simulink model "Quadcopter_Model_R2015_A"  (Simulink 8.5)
settings: Solver=ode45  SolverMode=SingleTasking  StartTime=0.0  StopTime=runtime  RelTol=1e-3
InitFcn:
  | clear mex
  | delete test_model_sfun.mexw64
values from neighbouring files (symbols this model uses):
  g = 9.81    [modelParameters.m]    (also in analyzeIMU_data.m = 9.8; getMomentOfInertia.m = 9.80665)
  height_controlled_o = dataStruct.RC_Throttle_Constant.data(1)    [modelParameters.m]
  If = 0.3836    [modelParameters.m]    (also in thrustDragConstantCalculations.m = [If0; If1; If2; If3]; Kd_error.m = I_0 * sign(rotor_speed_0) + I_1 * rotor_speed_0 + I_2 * roto)
  Jreq = 4.2012e-05    [modelParameters.m]
  Jxx = 0.0130    (= 0.013)    [modelParameters.m]
  Jyy = 0.0140    (= 0.014)    [modelParameters.m]
  Jzz = 0.0285    [modelParameters.m]
  Kd = 1.4852e-07    [modelParameters.m]    (also in calcDragConstant.m = ((A'*A)^-1)*A'*b; thrustDragConstantCalculations.m = calcDragConstant(data, Pmin, Pmax, Rm, Kv, Kq, If); Kd_error.m = 1.0317e-07)
  Kq = 96.3422    [modelParameters.m]    (also in thrustDragConstantCalculations.m; Kd_error.m)
  Kt = 1.2007e-05    [modelParameters.m]    (also in calcThrustConstant.m = ((A'*A)^(-1))*(A'*T); thrustDragConstantCalculations.m = calcThrustConstant(data))
  Kv = 96.3422    [modelParameters.m]    (also in thrustDragConstantCalculations.m; Kd_error.m)
  m = 1.140    (= 1.14)    [modelParameters.m]
  omega0_o = (sqrt(((height_controlled_o      - Pmin)/(Pmax - Pmin)* Vb - Rm * If) * 4 *      Rm * Kv^2 * Kq * Kd + 1) - 1) / (2 * Rm *       Kv * Kq * Kd)    [modelParameters.m]
  omega1_o = omega0_o    [modelParameters.m]
  omega2_o = omega0_o    [modelParameters.m]
  omega3_o = omega0_o    [modelParameters.m]
  pitch_o = pitch_measured_VRPN(1)    [modelParameters.m]
  pitchrate_o = (pitch_measured_VRPN(1) - pitch_measured_VRPN(2))/(time(1) - time(2))    [modelParameters.m]
  Pmax = 2e5    (= 200000)    [modelParameters.m]    (also in thrustDragConstantCalculations.m; Kd_error.m)
  Pmin = 1e5    (= 100000)    [modelParameters.m]    (also in thrustDragConstantCalculations.m; Kd_error.m)
  rhx = 0.16    [modelParameters.m]
  rhy = 0.16    [modelParameters.m]
  rhz = 0.03    [modelParameters.m]
  Rm = 0.2308    [modelParameters.m]    (also in thrustDragConstantCalculations.m; Kd_error.m)
  roll_o = roll_measured_VRPN(1)    [modelParameters.m]
  rollrate_o = (roll_measured_VRPN(1) - roll_measured_VRPN(2))/(time(1) - time(2))    [modelParameters.m]
  Tc = 0.04    [modelParameters.m]
  Tq = 0.005    [modelParameters.m]
  Vb = 11.4    [modelParameters.m]    (also in calcDragConstant.m = [data.(6); data.(6); data.(6); data.(6)]; Kd_error.m = data.(6))
  x_controlled_o = 0    [modelParameters.m]
  x_o = x_position(1)    [modelParameters.m]
  x_vel_o = (x_position(1) - x_position(2))/(time(1) - time(2))    [modelParameters.m]
  y_controlled_o = 0    [modelParameters.m]
  y_o = y_position(1)    [modelParameters.m]
  y_vel_o = (y_position(1) - y_position(2))/(time(1) - time(2))    [modelParameters.m]
  yaw_controlled_o = 0    [modelParameters.m]
  yaw_o = 0    [modelParameters.m]
  yawrate_o = 0    [modelParameters.m]
  z_o = z_position(1)    [modelParameters.m]
  z_vel_o = (z_position(1) - z_position(2))/(time(1) - time(2))    [modelParameters.m]
undefined symbols (not defined in the file or in its folder): DiscIntNeverNeededParam
libraries: simulink x12, vrlib x2
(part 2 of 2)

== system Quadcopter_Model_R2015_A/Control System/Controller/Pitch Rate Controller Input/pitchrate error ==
  From Workspace2 : FromWorkspace  VariableName=pitchrate_error  SampleTime=Tq
  pitchrate_error : Outport
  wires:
  From Workspace2/1 -> pitchrate_error/1

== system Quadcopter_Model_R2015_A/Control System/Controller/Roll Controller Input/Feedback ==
  roll_error_model : Inport
  roll_error : Outport
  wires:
  roll_error_model/1 -> roll_error/1

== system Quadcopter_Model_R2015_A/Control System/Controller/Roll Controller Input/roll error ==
  From Workspace4 : FromWorkspace  VariableName=roll_error  SampleTime=Tq
  roll_error : Outport
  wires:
  From Workspace4/1 -> roll_error/1

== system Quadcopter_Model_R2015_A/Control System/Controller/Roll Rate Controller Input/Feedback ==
  rollrate_error_model : Inport
  rollrate_error : Outport
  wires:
  rollrate_error_model/1 -> rollrate_error/1

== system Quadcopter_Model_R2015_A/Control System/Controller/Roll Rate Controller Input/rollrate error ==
  From Workspace5 : FromWorkspace  VariableName=rollrate_error  SampleTime=Tq
  rollrate_error : Outport
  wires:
  From Workspace5/1 -> rollrate_error/1

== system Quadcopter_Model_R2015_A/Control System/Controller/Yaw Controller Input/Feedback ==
  yaw_error_model : Inport
  yaw_error : Outport
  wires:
  yaw_error_model/1 -> yaw_error/1

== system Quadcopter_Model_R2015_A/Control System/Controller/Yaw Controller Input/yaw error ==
  From Workspace7 : FromWorkspace  VariableName=yaw_error  SampleTime=Tc
  yaw_error : Outport
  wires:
  From Workspace7/1 -> yaw_error/1

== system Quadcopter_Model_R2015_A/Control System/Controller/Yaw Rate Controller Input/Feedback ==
  yawrate_error_model : Inport
  yawrate_error : Outport
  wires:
  yawrate_error_model/1 -> yawrate_error/1

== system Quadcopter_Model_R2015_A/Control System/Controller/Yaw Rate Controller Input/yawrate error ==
  From Workspace8 : FromWorkspace  VariableName=yawrate_error  SampleTime=Tq
  yawrate_error : Outport
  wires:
  From Workspace8/1 -> yawrate_error/1

== matlab function Actuation/Gravity

 ==
function E_Fg = gravity(m, g)

E_Fg = [0; 0; m*g];

== matlab function Actuation/Lbe





 ==
function E_ro  = linear_body_earth_conversion(B_vo, euler_angles)

euler_rates = zeros(3,1);
E_ro = zeros(3,1);

phi = euler_angles(1);
theta = euler_angles(2);
psi = euler_angles(3);

Leb = [cos(theta)*cos(psi), sin(phi)*sin(theta)*cos(psi)-cos(phi)*sin(psi), cos(phi)*sin(theta)*cos(psi)+sin(phi)*sin(psi); ...
       cos(theta)*sin(psi), sin(phi)*sin(theta)*sin(psi)+cos(phi)*cos(psi), cos(phi)*sin(theta)*sin(psi)-sin(phi)*cos(psi); ...
           -sin(theta)    ,                sin(phi)*cos(theta)            ,                 cos(phi)*cos(theta)           ];

E_ro = Leb * B_vo;

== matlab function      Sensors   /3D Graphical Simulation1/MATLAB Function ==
function y = eigenaxis_ucart(u)


if abs(u(1))< 0.0001
    u(1) = 0.0001;
end

if abs(u(2))< 0.0001
    u(2) = 0.0001;
end

if abs(u(3))< 0.0001
    u(3) = 0.0001;
end

u = [ -u(1); -u(2); u(3) ];% [Pitch, Yaw, Roll] 

C11 = cos(u(2))*cos(u(3));
C12 = cos(u(2))*sin(u(3));
C13 = -sin(u(2));
C21 = sin(u(1))*sin(u(2))*cos(u(3))-cos(u(1))*sin(u(3));
C22 = sin(u(1))*sin(u(2))*sin(u(3))+cos(u(1))*cos(u(3));
C23 = sin(u(1))*cos(u(2));
C31 = cos(u(1))*sin(u(2))*cos(u(3))+sin(u(1))*sin(u(3));
C32 = cos(u(1))*sin(u(2))*sin(u(3))-sin(u(1))*cos(u(3));
C33 = cos(u(1))*cos(u(2));
    
theta = acos(0.5*(C11+C22+C33-1));

e = [C23-C32; C31-C13; C12-C21]/(2*sin(theta));
    
y = [e; theta];

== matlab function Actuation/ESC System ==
function Vb_eff   = ESC(P, Pmin, Pmax, Vb)

P1 = P(1);
P2 = P(2);
P3 = P(3);
P4 = P(4);

% Define u_Pi for each of the rotors, limiting it to be greater than 0
% u_P0 = (rotor_0_duty_cycle/100 - Pmin) / (Pmax - Pmin);
% u_P1 = (rotor_1_duty_cycle/100 - Pmin) / (Pmax - Pmin);
% u_P2 = (rotor_2_duty_cycle/100 - Pmin) / (Pmax - Pmin);
% u_P3 = (rotor_3_duty_cycle/100 - Pmin) / (Pmax - Pmin);
u_P0 = (P1 - Pmin) / (Pmax - Pmin);
u_P1 = (P2 - Pmin) / (Pmax - Pmin);
u_P2 = (P3 - Pmin) / (Pmax - Pmin);
u_P3 = (P4 - Pmin) / (Pmax - Pmin);


% Determine the effective battery voltage from each ESC
Vb_eff_0 = u_P0 * Vb;
Vb_eff_1 = u_P1 * Vb;
Vb_eff_2 = u_P2 * Vb;
Vb_eff_3 = u_P3 * Vb;
    
Vb_eff = [Vb_eff_0, Vb_eff_1, Vb_eff_2, Vb_eff_3];

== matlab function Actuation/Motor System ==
function w_dot = motor(Vb_eff, w, Rm, Kv, Kq, Kd, If, Jreq)

% Define each motors effective battery voltage
Vb_eff_0 = Vb_eff(1);
Vb_eff_1 = Vb_eff(2);
Vb_eff_2 = Vb_eff(3);
Vb_eff_3 = Vb_eff(4);

% Determine the angular velocity of each rotor from feedback
w_0 = w(1);
w_1 = w(2);
w_2 = w(3);
w_3 = w(4);

% Determine angular acceleration of each rotor
w_0_dot = 1/(Jreq*Rm*Kq) * Vb_eff_0 - 1/(Jreq*Rm*Kq*Kv) * w_0 - 1/(Jreq*Kq)*If - (Kd/Jreq) * w_0^2;
w_1_dot = 1/(Jreq*Rm*Kq) * Vb_eff_1 - 1/(Jreq*Rm*Kq*Kv) * w_1 - 1/(Jreq*Kq)*If - (Kd/Jreq) * w_1^2;
w_2_dot = 1/(Jreq*Rm*Kq) * Vb_eff_2 - 1/(Jreq*Rm*Kq*Kv) * w_2 - 1/(Jreq*Kq)*If - (Kd/Jreq) * w_2^2;
w_3_dot = 1/(Jreq*Rm*Kq) * Vb_eff_3 - 1/(Jreq*Rm*Kq*Kv) * w_3 - 1/(Jreq*Kq)*If - (Kd/Jreq) * w_3^2;

w_dot = [w_0_dot, w_1_dot, w_2_dot, w_3_dot];

== matlab function Actuation/Rotor System







 ==
function [B_omega_dot, B_vo_dot]= rotor(w_dot, w, B_Fg, B_omega, B_vo, m, Kt, Kd, rhx, rhy, rhz, Jreq, Jxx, Jyy, Jzz)

% Create J vector
J = [Jxx,  0 ,  0 ; ...
      0 , Jyy,  0 ; ...
      0 ,  0 , Jzz;];

% Create r_hi vector
rh_0 = [-rhx; rhy; -rhz];
rh_1 = [rhx; rhy; -rhz];
rh_2 = [-rhx; -rhy; -rhz];
rh_3 = [rhx; -rhy; -rhz];

% Define vector from body frame origin to center of mass
br_oc = [0; 0; 0];

% Define 3x3 Identity Matrix
I = eye(3);

% Create gamma vectors
gamma_Ti = [0; 0; -1];
gamma_omega_03 = [0; 0; 1];  %Rotors 0 and 3 use this gamma_omega vector
gamma_omega_12 = [0; 0; -1]; %Rotors 1 and 2 use this gamma_omega vector

% Define angular velocities for each rotor
w_0 = w(1);
w_1 = w(2);
w_2 = w(3);
w_3 = w(4);

% Define angular acceleration for each rotor
w_0_dot = w_dot(1);
w_1_dot = w_dot(2);
w_2_dot = w_dot(3);
w_3_dot = w_dot(4);

% Define the rotor force in the z-direction from each rotor
B_Fr_0 = Kt * w_0 * w_0 * gamma_Ti;
B_Fr_1 = Kt * w_1 * w_1 * gamma_Ti;
B_Fr_2 = Kt * w_2 * w_2 * gamma_Ti;
B_Fr_3 = Kt * w_3 * w_3 * gamma_Ti;

% Sum up the rotor forces in the z-direction from each vector to get the
% total body force in the z-direction
B_Fr = B_Fr_0 + B_Fr_1 + B_Fr_2 + B_Fr_3;

% Define the in-plane drag and induced torque produced by each rotor
 B_Q_d0 = -1 * Kd * w_0 * w_0 * gamma_omega_03;
 B_Q_d1 = -1 * Kd * w_1 * w_1 * gamma_omega_12;
 B_Q_d2 = -1 * Kd * w_2 * w_2 * gamma_omega_12;
 B_Q_d3 = -1 * Kd * w_3 * w_3 * gamma_omega_03;

% Sum up the total in-plane drag and induced torque to get the total
% in-plane drag and induced torque on the body
B_Q_d = B_Q_d0 + B_Q_d1 + B_Q_d2 + B_Q_d3;

% Define the force lever arm torque created from the force produced by each
% rotor in the z-direction
B_Q_F0 = cross( rh_0, B_Fr_0 );
B_Q_F1 = cross( rh_1, B_Fr_1 );
B_Q_F2 = cross( rh_2, B_Fr_2 );
B_Q_F3 = cross( rh_3, B_Fr_3 );

B_Q_F = B_Q_F0 + B_Q_F1 + B_Q_F2 + B_Q_F3;

%Define the change in angular momentum torque produced by each rotor 
B_Q_L0 = -1 * Jreq * ( cross(B_omega, w_0 * gamma_omega_03) + w_0_dot * gamma_omega_03 );
B_Q_L1 = -1 * Jreq * ( cross(B_omega, w_1 * gamma_omega_12) + w_1_dot * gamma_omega_12 ); 
B_Q_L2 = -1 * Jreq * ( cross(B_omega, w_2 * gamma_omega_12) + w_2_dot * gamma_omega_12 ); 
B_Q_L3 = -1 * Jreq * ( cross(B_omega, w_3 * gamma_omega_03) + w_3_dot * gamma_omega_03 );

% Sum up the total change in angular momentum torque produced by each rotor
B_Q_L = B_Q_L0 + B_Q_L1 + B_Q_L2 + B_Q_L3;

% Define the total rotor system torque as the sum of the in-plane drag and
% induced torque, force lever arm torque, and change in angular momentum
% torques
B_Q = B_Q_d + B_Q_F + B_Q_L;

% Define the body forces in the z-direction from each vector to get the
% total body force in the z-direction
B_F = B_Fr + B_Fg; 

% Define the body frame linear velocities
B_vo_dot = (m*I)^(-1) * ( B_F - cross( B_omega, m*(B_vo + cross(B_omega, br_oc)) ) );

% Define the body frame angular velocities
B_omega_dot = J ^(-1) * ( B_Q - cross(B_omega, J * B_omega) - cross(br_oc, B_F) );

== matlab function Actuation/Aeb














 ==
function euler_rates = angular_body_earth_conversion(B_omega, euler_angles)

phi = euler_angles(1);
theta = euler_angles(2);

Aeb = [1,  sin(phi)*tan(theta), cos(phi)*tan(theta); ...
       0,      cos(phi)       ,        -sin(phi)   ; ...
       0,  sin(phi)/cos(theta), cos(phi)/cos(theta)];

   
euler_rates = Aeb * B_omega;

== matlab function Actuation/Lbe

















 ==
function [B_Fg, B_g]  = linear_earth_body_conversion(E_Fg, euler_angles, m)

phi = euler_angles(1);
theta = euler_angles(2);
psi = euler_angles(3);

Lbe = [             cos(theta)*cos(psi)              ,          cos(theta)*sin(psi)                  ,     -sin(theta)    ; ...
       sin(phi)*sin(theta)*cos(psi)-cos(phi)*sin(psi), sin(phi)*sin(theta)*sin(psi)+cos(phi)*cos(psi), sin(phi)*cos(theta); ...
       cos(phi)*sin(theta)*cos(psi)+sin(phi)*sin(psi), cos(phi)*sin(theta)*sin(psi)-sin(phi)*cos(psi), cos(phi)*cos(theta)];

B_Fg = Lbe * E_Fg;

B_g = B_Fg/m;

== matlab function      Sensors   /IMU





/






 ==
function [accelReading,gyroReading] = idealIMU(B_vo_dot, B_vo, B_Omega, B_g, r_oc, g)
%#codegen

a = B_vo_dot + cross(B_Omega,B_vo); % body frame acceleration 

accelReading = (a - B_g)/g ; % accelerometer reading (ideal)

gyroReading = B_Omega ; % gyroscope reading (ideal) 

end

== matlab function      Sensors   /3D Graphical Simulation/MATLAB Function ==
function y = eigenaxis_ucart(u)


if abs(u(1))< 0.0001
    u(1) = 0.0001;
end

if abs(u(2))< 0.0001
    u(2) = 0.0001;
end

if abs(u(3))< 0.0001
    u(3) = 0.0001;
end

u = [ -u(1); -u(2); u(3) ];% [Pitch, Yaw, Roll] 

C11 = cos(u(2))*cos(u(3));
C12 = cos(u(2))*sin(u(3));
C13 = -sin(u(2));
C21 = sin(u(1))*sin(u(2))*cos(u(3))-cos(u(1))*sin(u(3));
C22 = sin(u(1))*sin(u(2))*sin(u(3))+cos(u(1))*cos(u(3));
C23 = sin(u(1))*cos(u(2));
C31 = cos(u(1))*sin(u(2))*cos(u(3))+sin(u(1))*sin(u(3));
C32 = cos(u(1))*sin(u(2))*sin(u(3))-sin(u(1))*cos(u(3));
C33 = cos(u(1))*cos(u(2));
    
theta = acos(0.5*(C11+C22+C33-1));

e = [C23-C32; C31-C13; C12-C21]/(2*sin(theta));
    
y = [e; theta];

== matlab function      Sensors   /Aeb









 ==
function euler_rates_IMU = angular_body_earth_conversion(gyro_reading, euler_angles_filtered)

phi = euler_angles_filtered(1);
theta = euler_angles_filtered(2);

Aeb = [1, sin(phi)*tan(theta), cos(phi)*tan(theta); ...
       0,     cos(phi)       ,        -sin(phi)   ; ...
       0,  sin(phi)/cos(theta), cos(phi)/cos(theta)];

   
euler_rates_IMU = Aeb * gyro_reading;

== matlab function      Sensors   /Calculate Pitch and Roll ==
function [accel_pitch, accel_roll] = getPitchAndRoll(accel_reading, accel_roll_prev)

mag = norm(accel_reading);

% x_accel = accel_reading(1)/mag;
% y_accel = accel_reading(2)/mag;
% z_accel = accel_reading(3)/mag;

x_accel = accel_reading(1);
y_accel = accel_reading(2);
z_accel = accel_reading(3);

accel_pitch = atan(x_accel/sqrt(y_accel^2 + z_accel^2));

%accel_roll = atan2( -y_accel,(sign(-z_accel)*sqrt(z_accel^2 + (1/100)*x_accel^2)) );

%accel_roll = atan2( -y_accel,(sign(-z_accel)*sqrt(z_accel^2 + x_accel^2)) );
accel_roll = atan( -y_accel/( sqrt(z_accel^2 + x_accel^2))  );

% unwrapped_roll = unwrap([accel_roll_prev accel_roll]);
% accel_roll = unwrapped_roll(2);

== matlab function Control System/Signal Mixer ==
function P  = signal_mixer(height_controlled, y_controlled, x_controlled, yaw_controlled)

controller_outputs = [ height_controlled; x_controlled; y_controlled; yaw_controlled ];
signal_mixer = [ 1, -1, -1, -1; ... 
                 1,  1, -1,  1; ...
                 1, -1,  1,  1; ...
                 1,  1,  1, -1 ];

% signal_mixer = [ 1,  1, -1, -1; ... 
%                  1, -1, -1,  1; ...
%                  1,  1,  1,  1; ...
%                  1, -1,  1, -1 ];
             
P = signal_mixer * controller_outputs;

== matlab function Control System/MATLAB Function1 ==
function [z_corr, y_cor, x_corr, yaw_corr, pid_y_out, pid_roll_out] = c_controller(set_x, set_y, set_z, set_yaw, ...
    cur_x, cur_y, cur_z, ...
    cur_phi, cur_theta, cur_psi, ...
    cur_phi_d, cur_theta_d, cur_psi_d, vrpn_id, Tc)

out_z = -1;
out_y = -1;
out_x = -1;
out_yaw = -1;
c_pid_y = -1;
c_pid_roll = -1;

coder.ceval('c_controller', vrpn_id, Tc, set_x, set_y, set_z, set_yaw, ...
                    cur_x, cur_y, cur_z, ...
                    cur_phi, cur_theta, cur_psi, ...
                    cur_phi_d, cur_theta_d, cur_psi_d, ...
                    coder.wref(out_z), coder.wref(out_y), coder.wref(out_x), coder.wref(out_yaw), ...
                    coder.wref(c_pid_y), coder.wref(c_pid_roll));

z_corr = out_z;
y_cor = out_y;
x_corr = out_x;
pid_y_out = c_pid_y;
pid_roll_out = c_pid_roll;
yaw_corr = out_yaw;

== matlab function      Sensors   /Aeb_c









1 ==
function euler_rates_IMU = angular_body_earth_conversion(gyro_reading, euler_angles_filtered)

phi = euler_angles_filtered(1);
theta = euler_angles_filtered(2);
psi = NaN;

phi_dot = -1;
theta_dot = -1;
psi_dot = -1;

p = gyro_reading(1);
q = gyro_reading(2);
r = gyro_reading(3);

coder.ceval( 'aeb_mat', p, q, r, phi, theta, psi, coder.wref(phi_dot), ...
    coder.wref(theta_dot), coder.wref(psi_dot) );

   
euler_rates_IMU = [phi_dot; theta_dot; psi_dot];

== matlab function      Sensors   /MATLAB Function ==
function euler_angles_IMU  = complimentaryFilterC(accel_pitch, accel_roll, euler_rates_gyro)

euler_x = euler_rates_gyro(1);
euler_y = euler_rates_gyro(2);

filtered_pitch = -1;
filtered_roll = -1;

coder.ceval('compl_filter', accel_pitch, accel_roll, euler_x, euler_y, ...
            coder.wref(filtered_pitch), coder.wref(filtered_roll));

euler_angles_IMU = [filtered_roll; filtered_pitch];

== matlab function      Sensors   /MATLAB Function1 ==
function [accel_pitch, accel_roll]  = angle_IMU_C(accel_reading)

accel_x = accel_reading(1);
accel_y = accel_reading(2);
accel_z = accel_reading(3);

calculated_pitch = -1;
calculated_roll = -1;

coder.ceval('angle_accel', accel_x, accel_y, accel_z, coder.wref(calculated_pitch), coder.wref(calculated_roll));

accel_pitch = calculated_pitch;
accel_roll = calculated_roll;

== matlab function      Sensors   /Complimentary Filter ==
%function euler_angles_IMU  = complimentaryFilter(accel_pitch, accel_roll, euler_angles_gyro, prev_euler_angles_IMU)
function euler_angles_IMU  = complimentaryFilter(accel_pitch, accel_roll, euler_rates_gyro, prev_euler_angles)

k_gyro = 0.98; 
k_accel = 1-k_gyro; 

Ts = 0.005; % 5 milliseconds

prev_phi = prev_euler_angles(1);
prev_theta = prev_euler_angles(2);

prev_phi_dot = euler_rates_gyro(1);
prev_theta_dot = euler_rates_gyro(2);

integrated_phi_gyro = Ts * prev_phi_dot + prev_phi;
integrated_theta_gyro = Ts * prev_theta_dot + prev_theta;

phi = k_gyro * integrated_phi_gyro + k_accel * accel_roll;
theta = k_gyro * integrated_theta_gyro + k_accel * accel_pitch;

euler_angles_IMU = [phi; theta];
